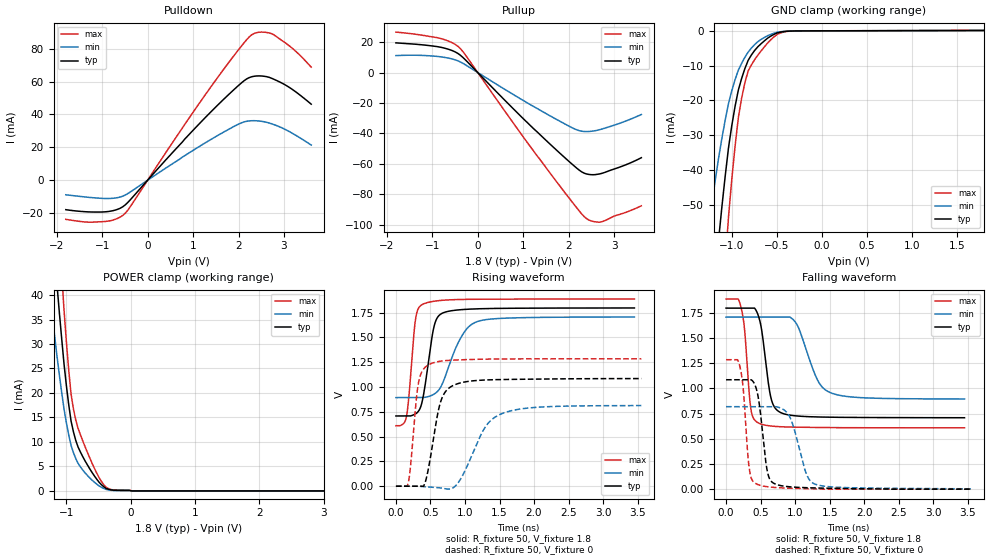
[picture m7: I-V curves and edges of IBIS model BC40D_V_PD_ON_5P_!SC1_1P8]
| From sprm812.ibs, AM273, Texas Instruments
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|   Model Cell BC40D_V_PD_ON_5P_!SC1_1P8
|BC40D_V_PD_ON_5P_!SC1_1P8
[Model]   BC40D_V_PD_ON_5P_!SC1_1P8
Model_type   I/O
Polarity   Non-Inverting
Enable   Active-Low
Vinl =  0.63
Vinh =  1.17
Cref =  15pF
Rref =  100.0000M
Vref =  0V
Vmeas =  0.9
C_comp   2.233931p   2.204415p   2.290246p
|[Input load] weak_pd_on
|[Output drive] fast
|[supplytol] 5
|[temp] ind
[Model Spec]
Vinl   0.63   0.5985   0.6615
Vinh   1.17   1.1115   1.2285
[Temperature Range]   25   125   -40
[Voltage Range]   1.8   1.71   1.89
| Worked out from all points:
|   slope of the pulldown table from 0 to 0.27 V, typ, clamps not added: 32.2 ohm
|   slope of the pullup table from 0 to 0.27 V, typ, clamps not added: 32.5 ohm
|   GND clamp passes 1 mA (typ) near -0.53 V on its own axis
|   POWER clamp passes 1 mA (typ) near -0.43 V on its own axis
|   rising waveform, R_fixture 50, V_fixture 1.8: 20-80 % time 141ps typ, 294ps min, 91.5ps max; typ from 0.708 V to 1.8 V
|   rising waveform, R_fixture 50, V_fixture 0: 20-80 % time 174ps typ, 350ps min, 104ps max; typ from 0 V to 1.09 V
|   falling waveform, R_fixture 50, V_fixture 1.8: 20-80 % time 128ps typ, 263ps min, 86.2ps max; typ from 1.8 V to 0.709 V
|   falling waveform, R_fixture 50, V_fixture 0: 20-80 % time 111ps typ, 195ps min, 82.5ps max; typ from 1.09 V to 0 V
| Nom Voltages:
|   VDD=1.1, VDDS=1.8, VDDS18=1.8, ESD_BIASFET=0, VSS=0, VSSS=0
| Min Voltages:
|   VDD=1.045, VDDS=1.71, VDDS18=1.71, ESD_BIASFET=0, VSS=0, VSSS=0
| Max Voltages:
|   VDD=1.16, VDDS=1.89, VDDS18=1.89, ESD_BIASFET=0, VSS=0, VSSS=0
[POWER_clamp]
|   voltage   I(typ)   I(min)   I(max)
-1.8V     158.9mA    112.5mA    219.9mA
-1.255V   60.04mA    40.04mA    85.04mA
-1.145V   41.99mA    27.45mA    59.9mA
-1.109V   36.4mA     23.66mA    51.97mA
-1.073V   31.03mA    20.08mA    44.3mA
-1.036V   25.91mA    16.71mA    36.9mA
-927.3mV  14.27mA    9.301mA    19.77mA
-854.5mV  10.33mA    6.623mA    14.48mA
-454.5mV  1.273mA    746.6uA    1.931mA
-309.1mV  221.6uA    137.5uA    298.5uA
18.18mV   0A         0A         0A
3.6V      0A         0A         0A
[Pulldown]
|   voltage   I(typ)   I(min)   I(max)
-1.8V     -17.92mA   -8.85mA    -23.8mA
-1.309V   -19.26mA   -10.37mA   -25.5mA
-927.3mV  -19.22mA   -11.12mA   -25.08mA
-654.5mV  -17.65mA   -10.56mA   -23.13mA
-490.9mV  -14.97mA   -8.985mA   -20.05mA
1.364V    40.78mA    24.32mA    55.69mA
2.073V    59.4mA     35mA       81.9mA
2.291V    62.96mA    36.2mA     88.48mA
2.509V    63.41mA    35.84mA    90.12mA
2.782V    61.38mA    33.82mA    88.42mA
3.218V    54.59mA    28.02mA    79.45mA
3.6V      46.26mA    21.39mA    68.79mA
[Pullup]
|   voltage   I(typ)   I(min)   I(max)
-1.8V     19.47mA    11.11mA    26.55mA
-818.2mV  16.61mA    10.32mA    22.37mA
-545.5mV  14.2mA     8.765mA    19.31mA
-381.8mV  11.35mA    6.927mA    15.71mA
1.255V    -37.58mA   -22.7mA    -52.59mA
2.127V    -61.49mA   -36.97mA   -86.91mA
2.291V    -65.3mA    -38.55mA   -92.97mA
2.4V      -66.65mA   -38.77mA   -96.07mA
2.564V    -67.08mA   -38.3mA    -97.93mA
2.727V    -66.24mA   -37.15mA   -97.99mA
3.273V    -60.4mA    -31.68mA   -91.65mA
3.6V      -55.92mA   -27.55mA   -87.52mA
[GND_clamp]
|   voltage   I(typ)   I(min)   I(max)
-1.8V     -270.2mA   -170.2mA   -430.1mA
-1.255V   -91.66mA   -55.91mA   -148.4mA
-1.145V   -59.91mA   -36.45mA   -97.1mA
-1.109V   -50.48mA   -30.83mA   -81.56mA
-1.073V   -41.73mA   -25.65mA   -67.06mA
-1.036V   -33.67mA   -20.93mA   -53.6mA
-927.3mV  -17.08mA   -11.35mA   -25.06mA
-854.5mV  -10.88mA   -7.624mA   -14.94mA
-781.8mV  -6.944mA   -4.956mA   -9.81mA
-636.4mV  -2.852mA   -1.883mA   -4.567mA
-381.8mV  -107.5uA   -92.09uA   -158.2uA
1.8V      101.9uA    59.12uA    150.8uA
[Ramp]
| variable   typ   min   max
dV/dt_f 0.66510514/0.13039257n 0.49951363/0.26900827n 0.77657515/87.836977p
dV/dt_r 0.66379743/0.17656601n 0.50939443/0.36426095n 0.78039524/0.10503855n
R_load = 50
[Rising Waveform]
R_fixture = 50
V_fixture = 1.8
V_fixture_min = 1.71
V_fixture_max = 1.89
|   time   V(typ)   V(min)   V(max)
0s        708.5mV    893.6mV    610.3mV
149.8ps   708.5mV    893.6mV    693.4mV
183.7ps   708.5mV    893.6mV    873.7mV
283.5ps   729.6mV    893.6mV    1.683V
386.4ps   874.1mV    894.9mV    1.834V
548.5ps   1.601V     927.1mV    1.865V
678.4ps   1.747V     1.043V     1.876V
933.5ps   1.78V      1.49V      1.883V
1.179ns   1.789V     1.661V     1.886V
3.453ns   1.798V     1.706V     1.887V
[Rising Waveform]
R_fixture = 50
V_fixture = 0
V_fixture_min = 0
V_fixture_max = 0
|   time   V(typ)   V(min)   V(max)
0s        0V         0V         0V
177.5ps   0V         0V         32.06mV
322.8ps   0V         0V         1.027V
401.5ps   0V         -4.657mV   1.183V
481.2ps   216.8mV    -8.352mV   1.228V
647.3ps   852mV      -17.62mV   1.261V
852.3ps   1.023V     -2.899mV   1.272V
1.28ns    1.071V     582.7mV    1.282V
1.512ns   1.076V     725.8mV    1.283V
3.554ns   1.086V     813.3mV    1.285V
[Falling Waveform]
R_fixture = 50
V_fixture = 1.8
V_fixture_min = 1.71
V_fixture_max = 1.89
|   time   V(typ)   V(min)   V(max)
0s        1.798V     1.708V     1.888V
212.8ps   1.798V     1.708V     1.817V
267.2ps   1.798V     1.708V     1.592V
357.7ps   1.798V     1.708V     804.9mV
465ps     1.728V     1.708V     658.8mV
646.9ps   915.8mV    1.708V     627.2mV
786.7ps   761.8mV    1.708V     619.9mV
1.018ns   727.3mV    1.645V     615.4mV
1.501ns   714.5mV    961.2mV    611.3mV
3.453ns   709.3mV    895.6mV    609.1mV
[Falling Waveform]
R_fixture = 50
V_fixture = 0
V_fixture_min = 0
V_fixture_max = 0
|   time   V(typ)   V(min)   V(max)
0s        1.086V     818.9mV    1.285V
199.2ps   1.086V     818.9mV    1.222V
249.5ps   1.086V     818.9mV    992mV
336.5ps   1.086V     818.9mV    203.3mV
437ps     999.5mV    818.9mV    53.09mV
592.7ps   195mV      818.9mV    24.49mV
707.8ps   52.57mV    818.9mV    16.66mV
926.3ps   23.14mV    712.2mV    9.557mV
1.286ns   12mV       50.67mV    2.853mV
3.554ns   0V         3.574mV    0V
